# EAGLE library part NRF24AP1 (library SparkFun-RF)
2.4GHz ANT IC Nordic Semiconductor 2.4GHz transceiver that implements the ANT protocol.
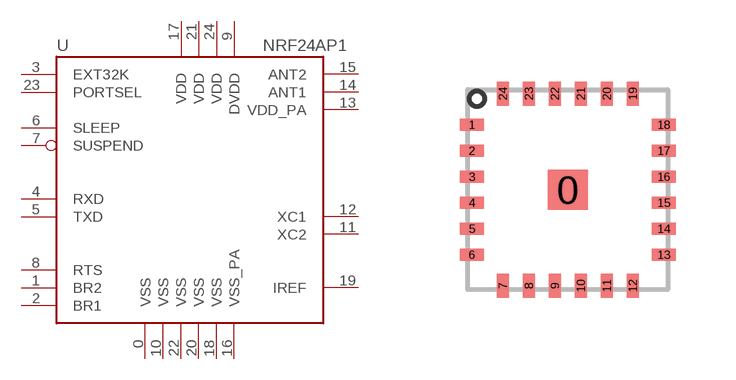
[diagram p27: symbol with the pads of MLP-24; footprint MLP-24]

Designator prefix U

## NRF24AP1SMD  [MLP-24]
0  VSS  out
1  BR2
2  BR1  in
3  EXT32K  in
4  RXD  in
5  TXD  out
6  SLEEP  in
7  SUSPEND  in
8  RTS  out
9  DVDD  pwr
10  VSS  pwr
11  XC2  in
12  XC1  in
13  VDD_PA  pwr
14  ANT1  out
15  ANT2  out
16  VSS_PA  pwr
17  VDD  pwr
18  VSS  pwr
19  IREF  in
20  VSS  pwr
21  VDD  pwr
22  VSS  pwr
23  PORTSEL  in
24  VDD  pwr

## Footprint MLP-24 (pad centres in mm)
smd 1 x 1: 0 0,0
smd 0.61 x 0.305: 1 -2.401,1.625; 2 -2.401,0.975; 3 -2.401,0.325; 4 -2.401,-0.325; 5 -2.401,-0.975; 6 -2.401,-1.625; 13 2.401,-1.625; 14 2.401,-0.975; 15 2.401,-0.325; 16 2.401,0.325; 17 2.401,0.975; 18 2.401,1.625
smd 0.305 x 0.61: 7 -1.625,-2.401; 8 -0.975,-2.401; 9 -0.325,-2.401; 10 0.325,-2.401; 11 0.975,-2.401; 12 1.625,-2.401; 19 1.625,2.401; 20 0.975,2.401; 21 0.325,2.401; 22 -0.325,2.401; 23 -0.975,2.401; 24 -1.625,2.401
